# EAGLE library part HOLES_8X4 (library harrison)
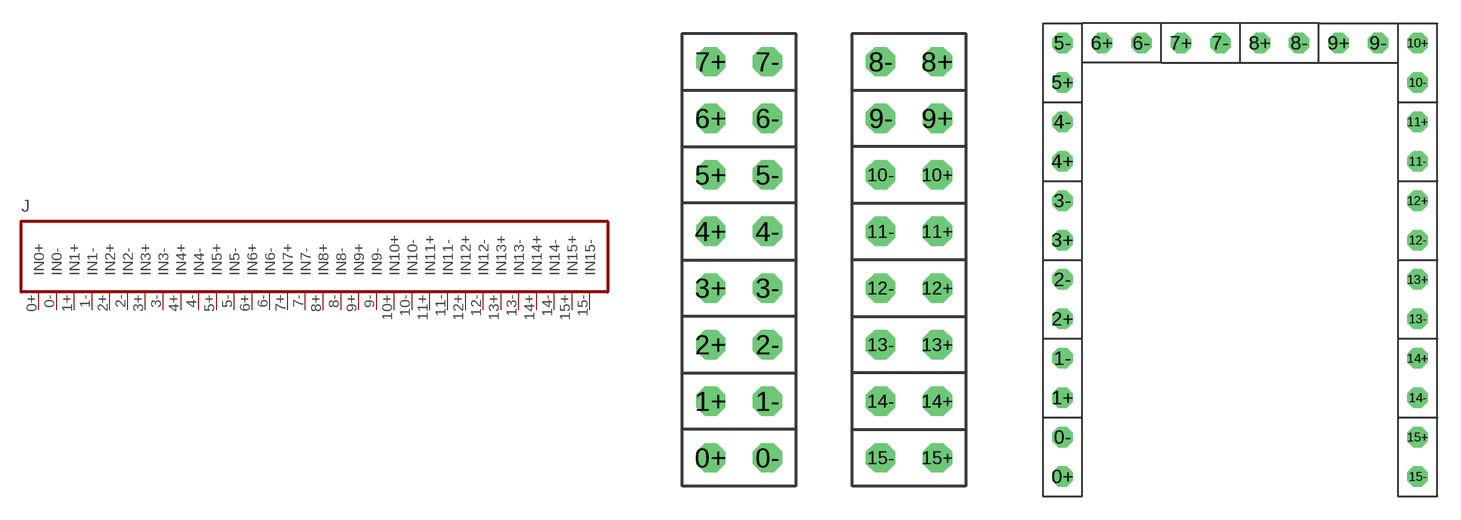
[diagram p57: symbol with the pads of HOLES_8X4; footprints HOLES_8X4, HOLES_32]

Designator prefix J

## HOLES_8X4  [HOLES_8X4]
0+  IN0+  pas
0-  IN0-  pas
1+  IN1+  pas
1-  IN1-  pas
2+  IN2+  pas
2-  IN2-  pas
3+  IN3+  pas
3-  IN3-  pas
4+  IN4+  pas
4-  IN4-  pas
5+  IN5+  pas
5-  IN5-  pas
6+  IN6+  pas
6-  IN6-  pas
7+  IN7+  pas
7-  IN7-  pas
8+  IN8+  pas
8-  IN8-  pas
9+  IN9+  pas
9-  IN9-  pas
10+  IN10+  pas
10-  IN10-  pas
11+  IN11+  pas
11-  IN11-  pas
12+  IN12+  pas
12-  IN12-  pas
13+  IN13+  pas
13-  IN13-  pas
14+  IN14+  pas
14-  IN14-  pas
15+  IN15+  pas
15-  IN15-  pas

## HOLES_8X4_HORSESHOE  [HOLES_32]
Pads as for HOLES_8X4

## Footprint HOLES_8X4 (pad centres in mm)
drill 0.813 octagon: 0+ -5.08,-8.89; 0- -2.54,-8.89; 1+ -5.08,-6.35; 1- -2.54,-6.35; 2+ -5.08,-3.81; 2- -2.54,-3.81; 3+ -5.08,-1.27; 3- -2.54,-1.27; 4+ -5.08,1.27; 4- -2.54,1.27; 5+ -5.08,3.81; 5- -2.54,3.81; 6+ -5.08,6.35; 6- -2.54,6.35; 7+ -5.08,8.89; 7- -2.54,8.89; 8+ 5.08,8.89; 8- 2.54,8.89; 9+ 5.08,6.35; 9- 2.54,6.35; 10+ 5.08,3.81; 10- 2.54,3.81; 11+ 5.08,1.27; 11- 2.54,1.27; 12+ 5.08,-1.27; 12- 2.54,-1.27; 13+ 5.08,-3.81; 13- 2.54,-3.81; 14+ 5.08,-6.35; 14- 2.54,-6.35; 15+ 5.08,-8.89; 15- 2.54,-8.89

## Footprint HOLES_32 (pad centres in mm)
drill 0.813 octagon: 0+ -11.43,-11.43; 0- -11.43,-8.89; 1+ -11.43,-6.35; 1- -11.43,-3.81; 2+ -11.43,-1.27; 2- -11.43,1.27; 3+ -11.43,3.81; 3- -11.43,6.35; 4+ -11.43,8.89; 4- -11.43,11.43; 5+ -11.43,13.97; 5- -11.43,16.51; 6+ -8.89,16.51; 6- -6.35,16.51; 7+ -3.81,16.51; 7- -1.27,16.51; 8+ 1.27,16.51; 8- 3.81,16.51; 9+ 6.35,16.51; 9- 8.89,16.51; 10+ 11.43,16.51; 10- 11.43,13.97; 11+ 11.43,11.43; 11- 11.43,8.89; 12+ 11.43,6.35; 12- 11.43,3.81; 13+ 11.43,1.27; 13- 11.43,-1.27; 14+ 11.43,-3.81; 14- 11.43,-6.35; 15+ 11.43,-8.89; 15- 11.43,-11.43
